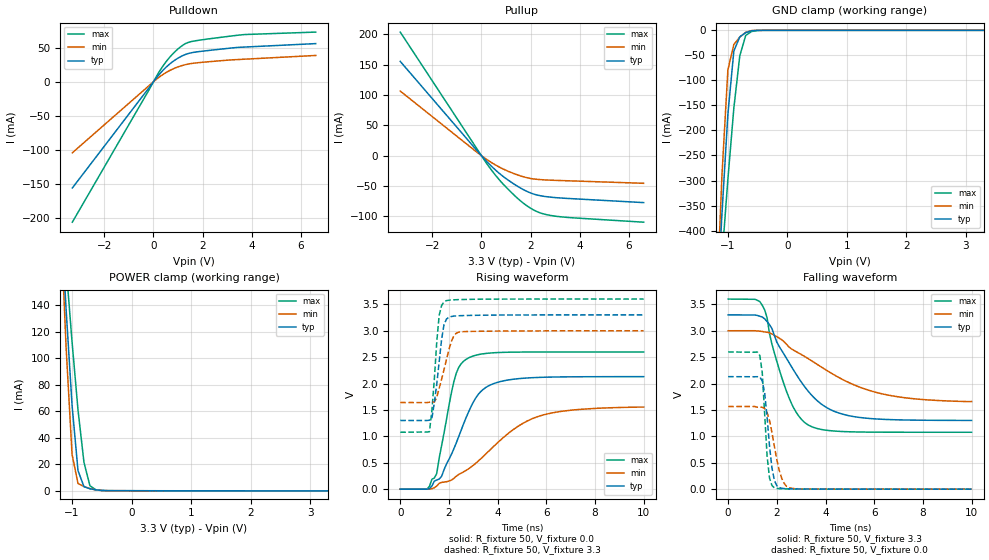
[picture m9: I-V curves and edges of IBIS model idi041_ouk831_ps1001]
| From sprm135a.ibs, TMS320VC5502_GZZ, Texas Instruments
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[Model]   idi041_ouk831_ps1001
|  I/O with pullup
Model_type   I/O
Vinh = 2.00
Vinl = 0.80
Enable   Active-Low
Polarity   Non-Inverting
| signals   A, GZ, Y
Vmeas = 1.5
|   typ   min   max
C_comp   1.7165p   1.6246p   1.9241p
|   typ   min   max
[Temperature Range]   25   -40   125
|   typ   min   max
[Voltage Range]   3.30V   3.00V   3.60V
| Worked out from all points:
|   slope of the pulldown table from 0 to 0.495 V, typ, clamps not added: 24 ohm
|   slope of the pullup table from 0 to 0.495 V, typ, clamps not added: 23.8 ohm
|   GND clamp passes 1 mA (typ) near -0.60 V on its own axis
|   POWER clamp passes 1 mA (typ) near -0.64 V on its own axis
|   rising waveform, R_fixture 50, V_fixture 0.0: 20-80 % time 1.22ns typ, 2.5ns min, 653ps max; typ from 0 V to 2.13 V
|   falling waveform, R_fixture 50, V_fixture 3.3: 20-80 % time 1.69ns typ, 3.01ns min, 997ps max; typ from 3.3 V to 1.3 V
|   rising waveform, R_fixture 50, V_fixture 3.3: 20-80 % time 303ps typ, 455ps min, 244ps max; typ from 1.3 V to 3.3 V
|   falling waveform, R_fixture 50, V_fixture 0.0: 20-80 % time 268ps typ, 408ps min, 208ps max; typ from 2.13 V to 0 V
[Pulldown]
|   Voltage   I(typ)   I(min)   I(max)
-3.3V     -155.6mA   -104.1mA   -205.6mA
200mV     9.244mA    5.866mA    12.7mA
600mV     24.13mA    15.28mA    33.3mA
800mV     29.87mA    18.87mA    41.37mA
1.1V      36.63mA    23.02mA    51.08mA
1.3V      39.97mA    25.04mA    55.82mA
1.6V      42.83mA    27mA       59.28mA
3.5V      50.44mA    32.65mA    68.4mA
6.6V      55.85mA    38.51mA    72.72mA
[GND_clamp]
|   Voltage   I(typ)   I(min)   I(max)
-3.3V     -5.888A    -7.654A    -4.434A
-1.2V     -591.9mA   -580.4mA   -622.5mA
-1.1V     -367mA     -290.3mA   -455.9mA
-1V       -167.6mA   -78.97mA   -297.5mA
-900mV    -41.5mA    -28.33mA   -155.5mA
-800mV    -12.94mA   -13.53mA   -50.92mA
-700mV    -4.664mA   -3.937mA   -10.14mA
-600mV    -901.7uA   -447.7uA   -2.289mA
-400mV    -4.618uA   -472.1nA   -49.36uA
3.3V      177.6pA    44.41pA    1.907uA
[Pullup]
|   Voltage   I(typ)   I(min)   I(max)
-3.3V     155.5mA    106.5mA    203.8mA
-200mV    9.303mA    6.23mA     12.42mA
300mV     -13.07mA   -8.543mA   -17.75mA
600mV     -24.68mA   -16mA      -33.64mA
900mV     -34.77mA   -22.33mA   -47.63mA
1.4V      -48.8mA    -30.78mA   -67.76mA
1.7V      -55.89mA   -34.78mA   -78.17mA
2V        -61.53mA   -37.68mA   -86.69mA
2.3V      -65.31mA   -39.22mA   -93.01mA
2.9V      -68.84mA   -40.61mA   -99.22mA
3.7V      -71.03mA   -41.73mA   -102.5mA
6.6V      -77.47mA   -45.64mA   -109.8mA
[POWER_clamp]
|   Voltage   I(typ)   I(min)   I(max)
-3.3V     2.113A     2.744A     1.594A
-1.2V     217.7mA    213mA      228.8mA
-1.1V     136.9mA    108.2mA    169.1mA
-1V       64.54mA    27.47mA    112.3mA
-900mV    15.16mA    5.443mA    60.93mA
-800mV    3.082mA    3.145mA    21.51mA
-700mV    1.489mA    1.661mA    3.764mA
-600mV    649.3uA    623.9uA    707.8uA
-500mV    185.1uA    140.5uA    173.8uA
3.3V      -108.3uA   -162.1uA   -68.06uA
[Ramp]
|   I(typ)   I(min)   I(max)
dV/dt_r   1.278/1.223n   0.933/2.496n   1.559/0.651n
dV/dt_f   1.199/1.693n   0.806/3.021n   1.513/0.996n
[Rising Waveform]
R_fixture = 50
V_fixture = 0.0
|  pu_on
|  TIME   V(typ)   V(min)   V(max)
0s        3nV        16nV       2nV
1.1ns     -143.1uV   -247.6uV   2.659mV
1.5ns     172.2mV    58.28mV    297.8mV
1.7ns     243.7mV    128.3mV    826.1mV
2.2ns     760.8mV    202mV      2.031V
2.4ns     992.5mV    277.9mV    2.303V
2.8ns     1.455V     383.5mV    2.484V
3.6ns     1.949V     704mV      2.574V
5.6ns     2.115V     1.366V     2.597V
10ns      2.13V      1.554V     2.598V
[Falling Waveform]
R_fixture = 50
V_fixture = 3.3
V_fixture_min = 3.0
V_fixture_max = 3.6
|  pd_on
|  TIME   V(typ)   V(min)   V(max)
0s        3.3V       3V         3.6V
1.4ns     3.261V     2.986V     3.483V
1.8ns     3.041V     2.939V     2.744V
2.4ns     2.475V     2.742V     1.849V
2.8ns     2.172V     2.603V     1.453V
3.3ns     1.848V     2.468V     1.212V
4.1ns     1.53V      2.234V     1.112V
5.1ns     1.379V     1.99V      1.085V
7ns       1.313V     1.748V     1.078V
10ns      1.302V     1.659V     1.078V
[Rising Waveform]
R_fixture = 50
V_fixture = 3.3
V_fixture_min = 3.0
V_fixture_max = 3.6
|  pd_off
|  TIME   V(typ)   V(min)   V(max)
0s        1.301V     1.641V     1.078V
1.2ns     1.306V     1.646V     1.089V
1.3ns     1.342V     1.649V     1.486V
1.5ns     1.987V     1.74V      2.787V
1.6ns     2.415V     1.912V     3.296V
1.7ns     2.838V     2.081V     3.478V
1.8ns     3.119V     2.265V     3.549V
2.1ns     3.27V      2.797V     3.583V
2.4ns     3.284V     2.974V     3.589V
10ns      3.3V       3V         3.6V
[Falling Waveform]
R_fixture = 50
V_fixture = 0.0
|  pu_off
|  TIME   V(typ)   V(min)   V(max)
0s        2.131V     1.565V     2.598V
1.3ns     2.125V     1.554V     2.531V
1.4ns     2.049V     1.551V     2.213V
1.5ns     1.826V     1.527V     1.419V
1.6ns     1.359V     1.451V     626.1mV
1.7ns     812.3mV    1.3V       208mV
1.9ns     163.6mV    806.3mV    24.86mV
2.2ns     16.78mV    207mV      7.277mV
2.6ns     6.083mV    16.64mV    3.36mV
10ns      2.403uV    67.96uV    1.39uV
